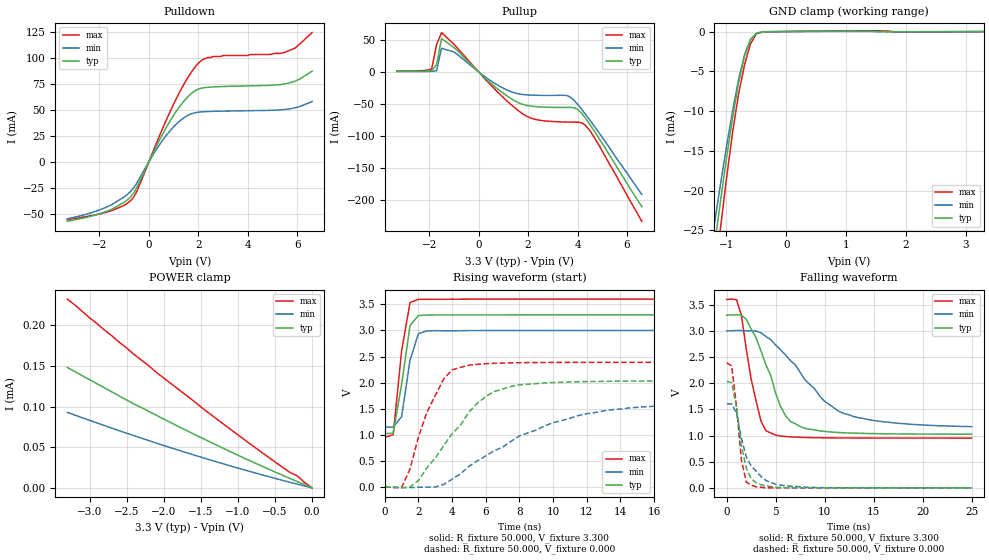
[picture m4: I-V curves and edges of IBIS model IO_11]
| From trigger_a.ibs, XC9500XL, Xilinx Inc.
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|   Model IO_11
[Model]   IO_11
Model_type   I/O
Polarity   Inverting
Enable   Active-High
Vinl =   0.800V
Vinh =   2.000V
Vmeas =   1.650V
Cref =  50.000pF
Rref =   1.000M
Vref =  0.000V
C_comp   6.700pF   5.700pF   7.600pF
[Temperature Range]   50.000   100.000   0.000
[Voltage Range]   3.300V   3.000V   3.600V
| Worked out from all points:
|   slope of the pulldown table from 0 to 0.495 V, typ, clamps not added: 20.7 ohm
|   slope of the pullup table from 0 to 0.495 V, typ, clamps not added: 27.8 ohm
|   GND clamp passes 1 mA (typ) near -0.59 V on its own axis
|   rising waveform, R_fixture 50.000, V_fixture 3.300: 20-80 % time 650ps typ, 615ps min, 600ps max; typ from 1.02 V to 3.3 V
|   rising waveform, R_fixture 50.000, V_fixture 0.000: 20-80 % time 2.98ns typ, 5.86ns min, 1.64ns max; typ from 0 V to 2.03 V
|   falling waveform, R_fixture 50.000, V_fixture 3.300: 20-80 % time 2.67ns typ, 5.37ns min, 1.56ns max; typ from 3.3 V to 1.02 V
|   falling waveform, R_fixture 50.000, V_fixture 0.000: 20-80 % time 1.06ns typ, 1.84ns min, 790ps max; typ from 2.03 V to 0 V
[Pulldown]
| voltage   I(typ)   I(min)   I(max)
-3.3V     -57.2mA    -54.8mA    -55.7mA
-1.7V     -47.57mA   -43.39mA   -48.32mA
-700mV    -32.66mA   -27.57mA   -36.39mA
-500mV    -25.26mA   -20.88mA   -29mA
300mV     14.82mA    11.72mA    17.61mA
900mV     40.85mA    30.95mA    50.29mA
1.6V      62.9mA     44.78mA    81.73mA
2.1V      70.46mA    47.8mA     96.79mA
3V        72.23mA    48.59mA    102mA
5.5V      74.68mA    50.15mA    105mA
5.9V      77.27mA    51.71mA    109mA
6.6V      86.93mA    57.76mA    124mA
[Pullup]
| voltage   I(typ)   I(min)   I(max)
-3.3V     899uA      569uA      1.459mA
-1.9V     1.866mA    805uA      4.44mA
-1.7V     11.19mA    1.78mA     42.55mA
-1.5V     52.16mA    36.93mA    61.56mA
-1V       38.26mA    31.19mA    43.28mA
700mV     -24.52mA   -19.08mA   -28.86mA
1.8V      -51.09mA   -35.45mA   -66.17mA
2.4V      -54.73mA   -36.71mA   -75.27mA
3.7V      -55.7mA    -39.34mA   -78.66mA
4V        -58.7mA    -50.64mA   -78.84mA
4.5V      -82.32mA   -75.47mA   -91.71mA
6.6V      -211mA     -192mA     -234mA
[GND_clamp]
| voltage   I(typ)   I(min)   I(max)
-3.3V     -155mA     -140mA     -172mA
-1.2V     -26.97mA   -24.12mA   -31.21mA
-1.1V     -21.35mA   -19.21mA   -24.73mA
-1V       -15.97mA   -14.5mA    -18.53mA
-900mV    -10.95mA   -10.08mA   -12.81mA
-800mV    -6.54mA    -6.125mA   -7.981mA
-700mV    -3.156mA   -2.96mA    -4.255mA
-600mV    -1.062mA   -1.009mA   -1.564mA
-500mV    -216uA     -233uA     -293uA
-400mV    -48.58uA   -49.49uA   -64.66uA
700mV     37.32uA    20.73uA    65.45uA
3.3V      1.628nA    6.9uA      -17.62uA
[POWER_clamp]
| voltage   I(typ)   I(min)   I(max)
-3.3V     148uA      92.8uA     232uA
-2.4V     103uA      64.12uA    164uA
-1.5V     61.88uA    37.81uA    99.54uA
-500mV    19.51uA    11.69uA    31.91uA
-300mV    11.57uA    6.9uA      19.07uA
-200mV    7.689uA    4.565uA    14.73uA
-100mV    4uA        2.274uA    6.481uA
0V        1.628nA    6.511nA    380pA
[Ramp]
| variable   typ   min   max
dV/dt_r   1.220/2.872n   0.961/5.818n   1.433/1.570n
dV/dt_f   1.365/2.644n   1.098/5.232n   1.589/1.447n
R_load = 50.000
[Rising Waveform]
R_fixture = 50.000
V_fixture = 3.300
V_fixture_min = 3.000
V_fixture_max = 3.600
L_fixture = 0.000H
C_fixture = 0.000F
| time   V(typ)   V(min)   V(max)
0s        1.023V     1.148V     951mV
500ps     1.029V     1.148V     1V
1ns       1.967V     1.346V     2.608V
1.5ns     3.093V     2.432V     3.534V
2ns       3.286V     2.939V     3.596V
2.5ns     3.295V     2.99V      3.596V
3ns       3.297V     2.996V     3.597V
25ns      3.3V       3V         3.6V
[Rising Waveform]
R_fixture = 50.000
V_fixture = 0.000
V_fixture_min = 0.000
V_fixture_max = 0.000
L_fixture = 0.000H
C_fixture = 0.000F
| time   V(typ)   V(min)   V(max)
0s        0V         0V         0V
1ns       -16.94mV   -12.49mV   -8.235mV
1.5ns     -699uV     -12.09mV   345mV
2.5ns     367mV      -2.934mV   1.429V
3.5ns     790mV      47.81mV    2.067V
4ns       1.021V     150mV      2.246V
6ns       1.733V     597mV      2.362V
8ns       1.957V     978mV      2.382V
13.5ns    2.026V     1.481V     2.388V
25ns      2.033V     1.6V       2.389V
[Falling Waveform]
R_fixture = 50.000
V_fixture = 3.300
V_fixture_min = 3.000
V_fixture_max = 3.600
L_fixture = 0.000H
C_fixture = 0.000F
| time   V(typ)   V(min)   V(max)
0s        3.3V       3V         3.6V
1ns       3.31V      3.009V     3.596V
1.5ns     3.3V       3.006V     3.296V
2.5ns     3.034V     3.002V     2.073V
3.5ns     2.617V     2.964V     1.272V
4ns       2.352V     2.893V     1.093V
6ns       1.381V     2.54V      981mV
8ns       1.137V     2.061V     962mV
13ns      1.045V     1.361V     953mV
25ns      1.025V     1.17V      951mV
[Falling Waveform]
R_fixture = 50.000
V_fixture = 0.000
V_fixture_min = 0.000
V_fixture_max = 0.000
L_fixture = 0.000H
C_fixture = 0.000F
| time   V(typ)   V(min)   V(max)
0s        2.033V     1.606V     2.389V
500ps     2.013V     1.606V     2.334V
1ns       1.543V     1.428V     1.557V
1.5ns     803mV      946mV      530mV
2ns       379mV      588mV      110mV
2.5ns     176mV      417mV      51.47mV
3ns       96.85mV    320mV      21.28mV
4ns       36.01mV    140mV      471uV
6ns       4.294mV    41.14mV    435uV
25ns      22.25uV    106uV      1.861uV
